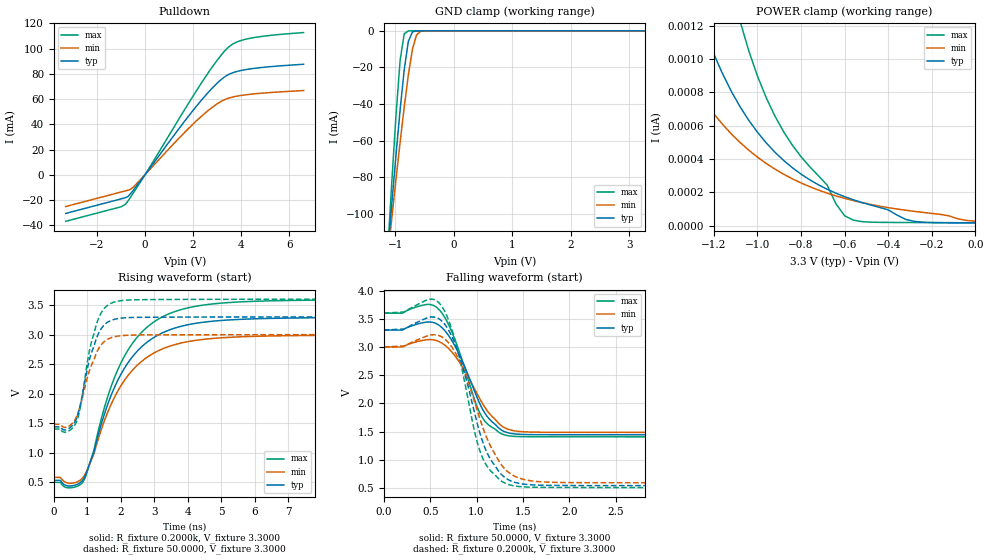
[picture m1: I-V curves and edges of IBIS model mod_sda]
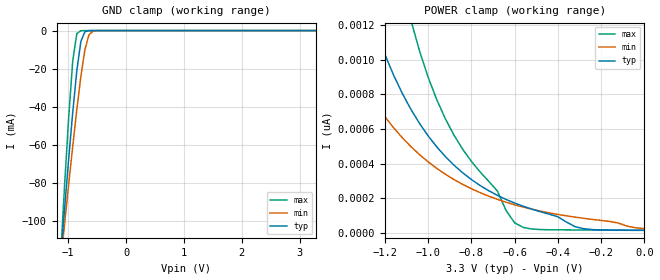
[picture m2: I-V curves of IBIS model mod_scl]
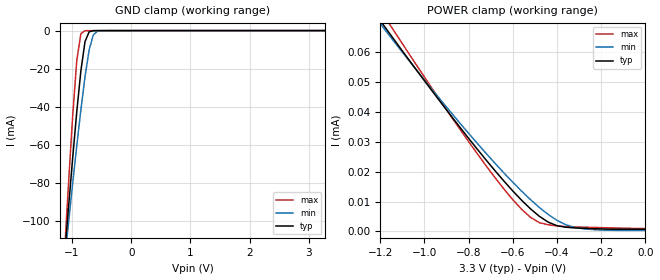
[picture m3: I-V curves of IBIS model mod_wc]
| IBIS (I/O, Buffer, Information, Specification) Model, officially
| electronic behavioral standard for Buffer structures of digital pins.
[IBIS ver]  4.0
[File name] m24m02e_3d3_dfn8.ibs
[File Rev]  1.0
[Date]   10 May 2023
[Source]   CAD & Design Services (Catania) - STMicroelectronics
[Notes]
   (Note1)  This IBIS model includes the DFN8 package parasitic data
   (Note2)  This IBIS model has some Notes about the non-monotonicity
   of the I-V curves, but they are not indicative of problems
   inside the model;
[Disclaimer]
   Customers are solely responsible for all aspects of their
   own product designs or applications using this IBIS Model.
   STMicroelectronics assumes no liability for Custmer Designs
   and applications associated to this IBIS Model.
   In the use of this IBIS Model Customer shall not modify,
   disassemble, alter this Model in whole or in part.
   If Customers do not accept these terms, the IBIS Model
   may not be used. For any problems or modifications please
   contact STMicroelectronics (www.st.com).
[Copyright] (c) 2023 STMicroelectronics
|   Component M24m02e
[Component] M24m02e
[Manufacturer] STMicroelectronics
[Package]
| variable  typ   min   max
R_pkg   0.0   0.0   0.0
L_pkg   0.0H   0.0H   0.0H
C_pkg   0.0F   0.0F   0.0F
[Pin]  signal_name   model_name   R_pin   L_pin   C_pin
1   DU   NC   0.0   0.0   0.0
2   E2   mod_en   0.0   0.0   0.0
3   E3   mod_en   0.0   0.0   0.0
4   VSS   GND   0.0   0.0   0.0
5   SDA   mod_sda   0.0   0.0   0.0
6   SCL   mod_scl   0.0   0.0   0.0
7   WC   mod_wc   0.0   0.0   0.0
8   VCC   POWER   0.0   0.0   0.0
[Package Model]  182694_DFN8   | also called 182694_MLP_2x3
[Define Package Model]  182694_DFN8
[Manufacturer]  STMicroelectronics
[OEM]  STMicroelectronics
[Description]  8 pin DFN8 2x3
[Number Of Pins]  8
[Pin Numbers]
|Pin Num   Terminal Name
1   | net1
2   | net2
3   | net3
4   | net4_GND
5   | net5
6   | net6
7   | net7
8   | net8_VDD
[Model Data]
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[End Model Data]
[End Package Model]
| Models and submodels in the file (4): mod_sda (I/O_open_drain), mod_scl (Input), mod_wc (Input), mod_en (Input)
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|   Model mod_sda
[Model]   mod_sda
Model_type I/O_open_drain
Polarity   Inverting
Enable   Active-High
Vinl   =   0.990V
Vinh   =   2.310V
Vmeas  =   1.650V
Cref   =   30pF
Rref   =   500
Vref   =   3.300V
C_comp   4.636pF   4.427pF   4.854pF
[Temperature Range]  25.0000   85.0000   -40.0000
[Voltage Range]   3.3000V   3.0000V   3.6000V
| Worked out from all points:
|   slope of the pulldown table from 0 to 0.495 V, typ, clamps not added: 38.6 ohm
|   GND clamp passes 1 mA (typ) near -0.72 V on its own axis
|   rising waveform, R_fixture 0.2000k, V_fixture 3.3000: 20-80 % time 1.3ns typ, 1.31ns min, 1.29ns max; typ from 0.534 V to 3.29 V
|   rising waveform, R_fixture 50.0000, V_fixture 3.3000: 20-80 % time 477ps typ, 497ps min, 452ps max; typ from 1.44 V to 3.3 V
|   falling waveform, R_fixture 50.0000, V_fixture 3.3000: 20-80 % time 300ps typ, 328ps min, 271ps max; typ from 3.3 V to 1.44 V
|   falling waveform, R_fixture 0.2000k, V_fixture 3.3000: 20-80 % time 291ps typ, 332ps min, 254ps max; typ from 3.3 V to 0.534 V
[Pulldown]
|Voltage   I(typ)   I(min)   I(max)
-3.3V     -30.7mA    -25.23mA   -36.95mA
-1V       -19.2mA    -13.73mA   -25.45mA
-800mV    -18.11mA   -12.73mA   -23.16mA
-700mV    -17.15mA   -12.23mA   -20.6mA
-500mV    -12.56mA   -10.11mA   -14.89mA
1.4V      36.22mA    28.71mA    43.89mA
2.3V      58.05mA    45.54mA    71.37mA
3V        72.6mA     56.2mA     90.74mA
3.5V      79.7mA     60.87mA    101.6mA
3.9V      82.29mA    62.6mA     105.9mA
4.4V      84.03mA    63.87mA    108.4mA
6.6V      87.65mA    66.78mA    112.8mA
[GND_clamp]
|Voltage   I(typ)   I(min)   I(max)
-3.3V     -1.01A     -814.9mA   -1.404A
-1.13V    -120.1mA   -122.5mA   -118.8mA
-1.06V    -93.42mA   -101.5mA   -81.03mA
-990mV    -67.49mA   -80.83mA   -45.6mA
-920mV    -42.94mA   -60.76mA   -15.96mA
-850mV    -21.15mA   -41.63mA   -1.606mA
-780mV    -5.768mA   -24.18mA   -63.74uA
-710mV    -616.4uA   -10.08mA   -4.14uA
-640mV    -45.34uA   -2.266mA   -227.5nA
-570mV    -3.307uA   -288.2uA   -7.345nA
3.28V     15.71pA    85.37pA    15.34pA
[POWER_clamp]
|Voltage   I(typ)   I(min)   I(max)
-3.28V    8.108uA    4.441uA    13.9uA
-1.44V    2.157nA    1.226nA    5.11nA
-1.4V     1.906nA    1.108nA    4.359nA
-1.24V    1.164nA    741.3pA    2.31nA
-1.16V    911.1pA    607.7pA    1.684nA
-1.08V    714pA      499.1pA    1.229nA
-960mV    496.8pA    373.1pA    768.5pA
-880mV    391.1pA    308.5pA    563.5pA
-680mV    217.9pA    194.7pA    242.9pA
-600mV    173.5pA    163.3pA    59.05pA
-280mV    25.23pA    85.37pA    18.25pA
0V        15.81pA    26.21pA    16.88pA
[Ramp]
| variable   typ   min   max
dV/dt_r   1.1161/0.5213n   0.9100/0.5262n   1.3183/0.5287n
dV/dt_f   1.1164/0.3342n   0.9103/0.3515n   1.3185/0.3191n
R_load = 50.0000
[Rising Waveform]
R_fixture= 0.2000k
V_fixture= 3.3000
V_fixture_min= 3.0000
V_fixture_max= 3.6000
|time   V(typ)   V(min)   V(max)
0s        533.7mV    584.1mV    499.5mV
490ps     438.6mV    483.8mV    407.8mV
890ps     559.8mV    595.1mV    523.4mV
1.19ns    1.001V     969mV      1.029V
1.59ns    1.786V     1.657V     1.913V
1.97ns    2.29V      2.101V     2.478V
2.53ns    2.741V     2.5V       2.98V
3.19ns    3.014V     2.743V     3.283V
4.98ns    3.238V     2.944V     3.531V
10ns      3.292V     2.992V     3.592V
[Rising Waveform]
R_fixture= 50.0000
V_fixture= 3.3000
V_fixture_min= 3.0000
V_fixture_max= 3.6000
|time   V(typ)   V(min)   V(max)
0s        1.439V     1.483V     1.402V
370ps     1.389V     1.431V     1.352V
670ps     1.572V     1.601V     1.516V
810ps     1.86V      1.839V     1.826V
1.07ns    2.584V     2.399V     2.742V
1.27ns    2.93V      2.681V     3.167V
1.47ns    3.141V     2.861V     3.415V
1.77ns    3.251V     2.957V     3.543V
2.67ns    3.292V     2.994V     3.591V
10ns      3.299V     2.999V     3.599V
[Falling Waveform]
R_fixture= 50.0000
V_fixture= 3.3000
V_fixture_min= 3.0000
V_fixture_max= 3.6000
|time   V(typ)   V(min)   V(max)
0s        3.3V       3V         3.6V
200ps     3.3V       3V         3.6V
470ps     3.442V     3.129V     3.755V
590ps     3.391V     3.1V       3.672V
750ps     3.067V     2.877V     3.202V
990ps     2.165V     2.22V      2.007V
1.05ns    1.94V      2.034V     1.78V
1.15ns    1.699V     1.797V     1.59V
1.35ns    1.473V     1.535V     1.423V
10ns      1.439V     1.483V     1.402V
[Falling Waveform]
R_fixture= 0.2000k
V_fixture= 3.3000
V_fixture_min= 3.0000
V_fixture_max= 3.6000
|time   V(typ)   V(min)   V(max)
0s        3.3V       3V         3.6V
500ps     3.529V     3.21V      3.848V
610ps     3.481V     3.192V     3.755V
790ps     2.956V     2.842V     2.978V
970ps     1.885V     2.069V     1.56V
1.05ns    1.394V     1.654V     1.09V
1.23ns    813.8mV    1.005V     674.4mV
1.39ns    609.4mV    724.7mV    539.7mV
1.95ns    542.2mV    594.6mV    507.5mV
10ns      534.5mV    585mV      500.1mV
|   Model mod_scl
[Model]   mod_scl
Model_type Input
Vinl   =   0.990V
Vinh   =   2.310V
C_comp   3.063pF   2.925pF   3.207pF
[Temperature Range]  25.0000   85.0000   -40.0000
[Voltage Range]   3.3000V   3.0000V   3.6000V
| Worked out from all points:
|   GND clamp passes 1 mA (typ) near -0.72 V on its own axis
[GND_clamp]
|Voltage   I(typ)   I(min)   I(max)
-3.3V     -1.01A     -814.9mA   -1.404A
-1.13V    -120.1mA   -122.5mA   -118.8mA
-1.06V    -93.42mA   -101.5mA   -81.03mA
-990mV    -67.49mA   -80.83mA   -45.6mA
-920mV    -42.94mA   -60.76mA   -15.96mA
-850mV    -21.15mA   -41.63mA   -1.606mA
-780mV    -5.768mA   -24.18mA   -63.74uA
-710mV    -616.4uA   -10.08mA   -4.14uA
-640mV    -45.34uA   -2.266mA   -227.5nA
-570mV    -3.307uA   -288.2uA   -7.345nA
3.28V     15.71pA    85.37pA    15.34pA
[POWER_clamp]
|Voltage   I(typ)   I(min)   I(max)
-3.28V    8.108uA    4.441uA    13.9uA
-1.44V    2.157nA    1.226nA    5.11nA
-1.4V     1.906nA    1.108nA    4.359nA
-1.24V    1.164nA    741.3pA    2.31nA
-1.16V    911.1pA    607.7pA    1.684nA
-1.08V    714pA      499.1pA    1.229nA
-960mV    496.8pA    373.1pA    768.5pA
-880mV    391.1pA    308.5pA    563.5pA
-680mV    217.9pA    194.7pA    242.9pA
-600mV    173.5pA    163.3pA    59.05pA
-280mV    25.23pA    85.37pA    18.25pA
0V        15.81pA    26.21pA    16.88pA
|   Model mod_wc
[Model]   mod_wc
Model_type Input
Vinl   =   0.990V
Vinh   =   2.310V
C_comp   3.063pF   2.925pF   3.207pF
[Temperature Range]  25.0000   85.0000   -40.0000
[Voltage Range]   3.3000V   3.0000V   3.6000V
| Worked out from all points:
|   GND clamp passes 1 mA (typ) near -0.72 V on its own axis
[GND_clamp]
|Voltage   I(typ)   I(min)   I(max)
-3.3V     -1.01A     -814.9mA   -1.404A
-1.13V    -120.1mA   -122.5mA   -118.8mA
-1.06V    -93.42mA   -101.5mA   -81.03mA
-990mV    -67.49mA   -80.83mA   -45.61mA
-920mV    -42.94mA   -60.76mA   -15.97mA
-850mV    -21.16mA   -41.63mA   -1.619mA
-780mV    -5.775mA   -24.18mA   -80.07uA
-710mV    -627.7uA   -10.09mA   -20.56uA
-640mV    -57.65uA   -2.273mA   -14.18uA
-570mV    -14.59uA   -297.1uA   -11.18uA
3.28V     12.26uA    11.36uA    14.65uA
[POWER_clamp]
|Voltage   I(typ)   I(min)   I(max)
-3.28V    304.1uA    290.5uA    326.2uA
-1.2V     70.66uA    69.64uA    74.29uA
-1.16V    66.58uA    65.8uA     69.73uA
-1.12V    62.53uA    61.99uA    65.2uA
-880mV    38.8uA     39.9uA     38.62uA
-680mV    20.32uA    22.8uA     17.99uA
-600mV    13.57uA    16.49uA    10.64uA
-520mV    7.592uA    10.68uA    4.744uA
-440mV    3.142uA    5.703uA    2.261uA
-400mV    1.933uA    3.725uA    1.867uA
-320mV    1.205uA    1.376uA    1.523uA
0V        716nA      355.6nA    974.2nA
